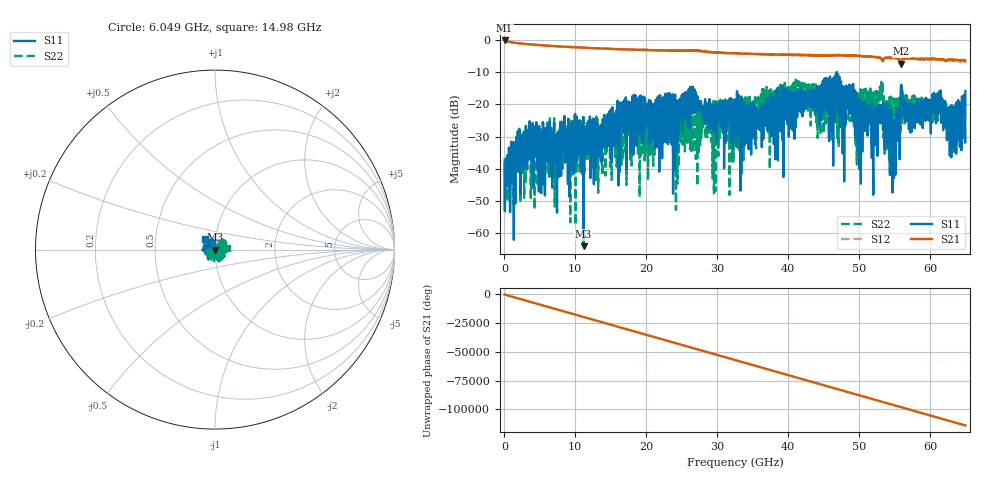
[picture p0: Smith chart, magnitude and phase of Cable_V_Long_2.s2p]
! Created Tue Jul 15 18:11:16 2008
# hz S ma R 50
! 2 Port Network Data from blockName block
! freq  magS11  angS11  magS21  angS21  magS12  angS12  magS22  angS22
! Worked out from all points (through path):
!   1601 points, 40 MHz to 65 GHz, reference 50 ohm
!   highest |S21| = -0.17 dB at 40 MHz (marker M1); lowest = -7.3 dB at 55.95 GHz (marker M2)
!   lowest |S11| = -63.9 dB at 11.16 GHz (marker M3), VSWR 1.00, Z = 50.1 + j0.035 ohm
!   |S11| at or under -10 dB: start of sweep to 46.85 GHz; 46.85 GHz to end of sweep
!   |S22| runs from -57.4 to -12.0 dB; largest |S21 - S12| = 0.058
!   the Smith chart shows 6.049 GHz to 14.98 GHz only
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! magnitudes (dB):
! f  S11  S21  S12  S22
! 40 MHz  -38.2  -0.2  -0.2  -36.7
! 486.6 MHz  -44.4  -0.5  -0.5  -42.5
! 3.572 GHz  -25.2  -1.4  -1.4  -26.5
! 7.389 GHz  -39.6  -2.0  -2.0  -31.9
! 10.27 GHz  -33.6  -2.3  -2.3  -32.7
! 10.88 GHz  -29.1  -2.4  -2.4  -30.0
! 11.16 GHz  -63.9  -2.4  -2.4  -28.5
! 16.65 GHz  -23.1  -2.9  -2.9  -20.9
! 21.72 GHz  -21.8  -3.2  -3.2  -25.1
! 26.47 GHz  -22.3  -3.4  -3.3  -22.2
! 32.52 GHz  -30.1  -4.1  -4.1  -31.1
! 43.36 GHz  -15.3  -4.7  -4.8  -18.7
! 46.77 GHz  -20.4  -4.7  -4.7  -25.7
! 49.82 GHz  -23.3  -5.0  -4.9  -17.8
! 53.06 GHz  -20.3  -5.7  -5.6  -18.4
! 54.2 GHz  -24.6  -5.5  -5.5  -22.1
! 55.05 GHz  -32.7  -5.6  -5.5  -25.1
! 55.95 GHz  -13.9  -7.3  -7.3  -15.5
! 57.33 GHz  -24.9  -5.8  -5.6  -19.4
! 61.22 GHz  -19.6  -6.1  -6.0  -18.5
! 63.42 GHz  -34.7  -6.2  -6.6  -22.0
! 65 GHz  -15.8  -6.4  -7.2  -23.5
